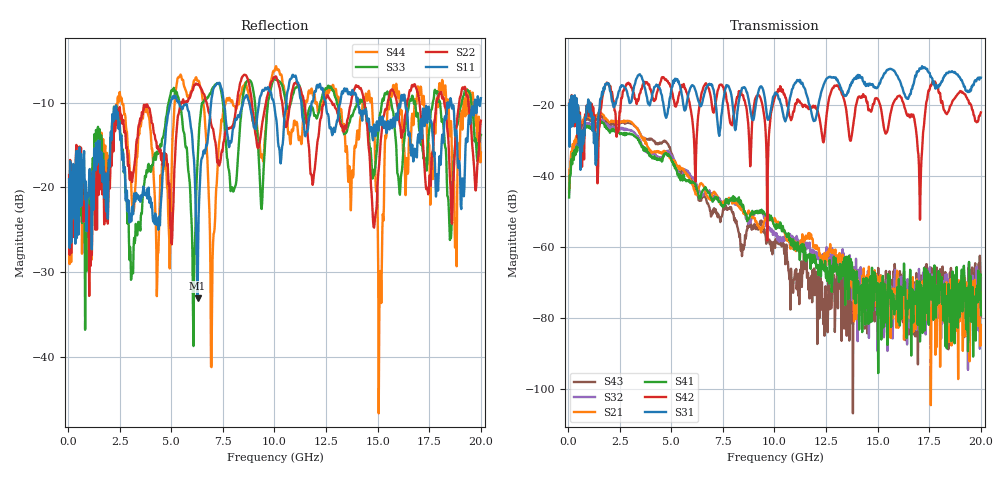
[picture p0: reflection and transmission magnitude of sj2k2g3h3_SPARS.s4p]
! FILE: E:\users\goganessyan\GBX_Backplane\FR408_backplane\1m_INBOUND_FEXT\sj2k2g3h3_SPARS.s4p
# MHZ S RI R 50.00
! FREQ  S11  S12  S13  S14
!  S21  S22  S23  S24
!  S31  S32  S33  S34
!  S41  S42  S43  S44
!  REAL  IMAG  REAL  IMAG  REAL  IMAG  REAL  IMAG
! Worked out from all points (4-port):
!   799 points, 50 MHz to 20 GHz, reference 50 ohm
!   strongest paths, dB at 50 MHz, 5.025 GHz, 10.03 GHz, 15.03 GHz, 20 GHz:
!     S31: -19.8, -15.0, -16.6, -14.8, -12.3
!     S42: -19.6, -16.1, -17.7, -18.5, -22.1
!     S41: -46.1, -35.9, -54.5, -95.7, -79.3
!     S21: -43.7, -35.8, -52.5, -75.2, -82.1
!     S32: -44.7, -34.2, -56.6, -73.0, -68.8
!     S43: -43.5, -34.2, -60.3, -66.0, -79.8
!   lowest |S11| = -33.1 dB at 6.275 GHz (marker M1), VSWR 1.05, Z = 49.8 - j2.19 ohm
!   |S11| at or under -10 dB: start of sweep to 4.965 GHz; 14.04 GHz to 16.11 GHz (2.067 GHz wide, 13.7 % of centre); 16.33 GHz to 18.37 GHz (2.04 GHz wide, 11.8 % of centre)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
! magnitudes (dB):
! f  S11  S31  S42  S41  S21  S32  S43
! 50 MHz  -19.0  -19.8  -19.6  -46.1  -43.7  -44.7  -43.5
! 6.275 GHz  -33.1  -18.0  -25.0  -44.4  -44.7  -43.1  -45.5
! 6.95 GHz  -9.5  -14.5  -19.2  -46.6  -45.7  -45.7  -50.9
! 8.55 GHz  -9.5  -15.0  -18.6  -50.0  -49.9  -50.7  -59.7
! 15.12 GHz  -11.7  -13.7  -20.1  -77.1  -68.1  -72.8  -79.5
! 15.7 GHz  -13.0  -10.0  -20.5  -77.5  -80.4  -85.7  -77.8
! 20 GHz  -9.5  -12.3  -22.1  -79.3  -82.1  -68.8  -79.8
